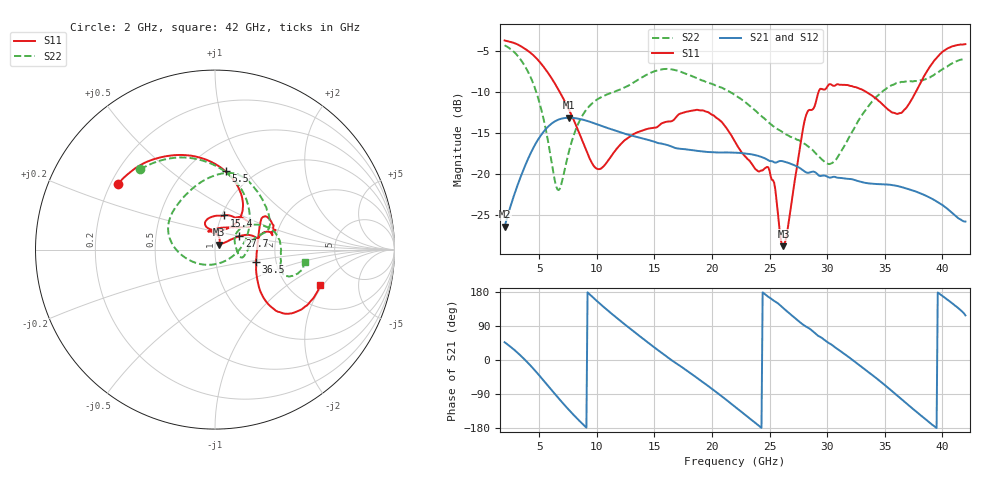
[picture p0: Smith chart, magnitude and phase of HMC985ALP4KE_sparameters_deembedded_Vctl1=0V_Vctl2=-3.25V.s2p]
!s2p File: Measurements: S11, S21, S12, S22
# GHz S dB R 50.0
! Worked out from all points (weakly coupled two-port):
!   401 points, 2 GHz to 42 GHz, reference 50 ohm
!   highest |S21| = -13.14 dB at 7.6 GHz (marker M1); lowest = -26.4 dB at 2 GHz (marker M2)
!   lowest |S11| = -28.8 dB at 26.2 GHz (marker M3), VSWR 1.08, Z = 52.3 + j2.93 ohm
!   |S11| at or under -10 dB: 6.789 GHz to 29.25 GHz (22.46 GHz wide, 125 % of centre); 33.41 GHz to 37.69 GHz (4.287 GHz wide, 12.1 % of centre)
!   |S22| runs from -22.0 to -4.3 dB; largest |S21 - S12| = 0.00069
!   S11 on the Smith chart (normalised r, x): 2 GHz: 0.23, +0.29; 5.5 GHz: 0.75, +0.81; 15.4 GHz: 1.03, +0.41; 27.7 GHz: 1.30, +0.20; 36.5 GHz: 1.57, -0.23; 42 GHz: 2.93, -1.90
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2  -3.70 146.2  -26.43 46.9  -26.43 46.9  -4.28 133.0
3.6  -4.56 118.9  -19.61 5.5  -19.62 5.5  -6.47 91.5
4.6  -5.64 100.0  -16.54 -26.5  -16.53 -26.5  -9.39 60.1
5.5  -7.13 82.3  -14.65 -58.3  -14.66 -58.4  -14.06 24.4
6.6  -9.53 63.6  -13.41 -98.0  -13.40 -98.0  -21.91 -65.3
7.6  -12.20 53.0  -13.14 -132.3  -13.15 -132.3  -17.17 -150.1
8.7  -15.80 53.9  -13.34 -166.8  -13.34 -166.8  -12.99 177.6
10.2  -19.41 87.8  -14.03 150.6  -14.00 150.6  -10.77 154.4
12.5  -15.81 109.9  -15.12 92.3  -15.09 92.3  -9.39 121.7
15.4  -14.10 75.0  -16.25 24.2  -16.26 24.2  -7.30 81.4
19.2  -12.24 33.6  -17.26 -58.1  -17.26 -58.1  -8.60 40.6
22  -16.04 51.8  -17.40 -123.3  -17.42 -123.3  -10.36 19.4
24.9  -19.20 104.2  -18.34 166.5  -18.31 166.5  -13.66 11.0
26.2  -28.82 50.7  -18.47 136.7  -18.49 136.7  -14.97 -3.3
27.7  -16.23 28.9  -19.35 98.2  -19.34 98.2  -16.02 -16.0
28.7  -12.16 12.8  -19.73 77.4  -19.73 77.4  -17.03 -14.6
30.6  -9.25 19.7  -20.35 35.5  -20.36 35.5  -18.47 23.0
33.2  -9.83 34.3  -21.06 -23.0  -21.05 -23.0  -12.47 35.2
35.4  -12.24 11.8  -21.31 -76.2  -21.30 -76.3  -9.35 17.5
36.5  -12.49 -16.6  -21.62 -104.6  -21.63 -104.6  -8.76 7.4
39.5  -5.84 -43.5  -23.36 -179.5  -23.33 -179.5  -7.68 -19.9
42  -4.15 -18.7  -25.82 117.8  -25.79 117.8  -5.94 -8.1
